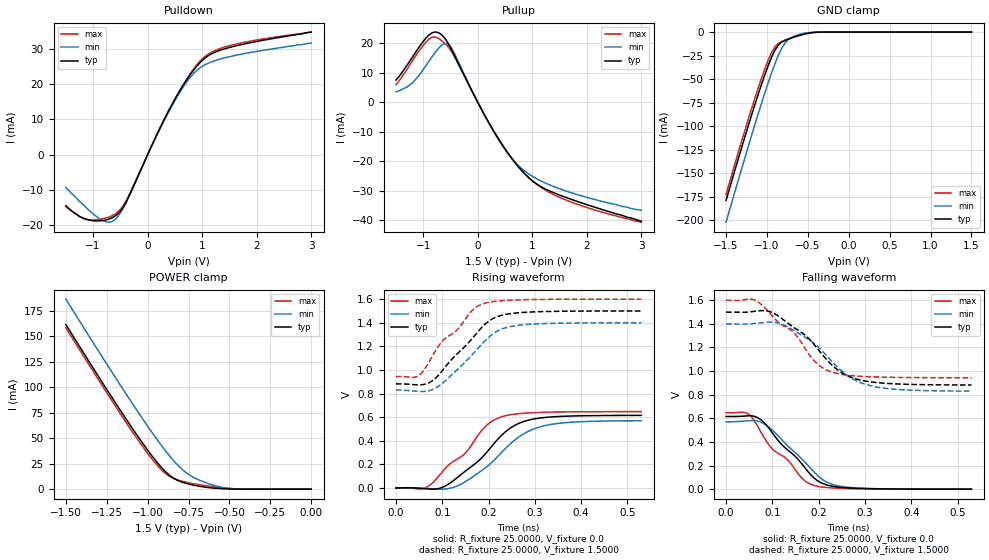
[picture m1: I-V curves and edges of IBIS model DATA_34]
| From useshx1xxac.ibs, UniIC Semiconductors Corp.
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|When TDQS is enabled, NU_TDQS is a output with terminal resistance;
|When TDQS is disabled, NU_TDQS is a DM;
|   Model DATA_34
[Model]  DATA_34
Model_type   I/O
Polarity   Non-Inverting
Enable   Active-High
Vinl =   0.600000V
Vinh =   0.900000V
Vmeas =   0.750000V
Rref =   25.0000000
Vref =   0.7500000V
C_comp   1.3900pF   1.3640pF   1.5600pF
[Temperature Range]   25.0000   95.0000   0.0
[Voltage Range]   1.5000V   1.4000V   1.6000V
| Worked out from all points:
|   slope of the pulldown table from 0 to 0.225 V, typ, clamps not added: 29.8 ohm
|   slope of the pullup table from 0 to 0.225 V, typ, clamps not added: 29.6 ohm
|   GND clamp passes 1 mA (typ) near -0.48 V on its own axis
|   POWER clamp passes 1 mA (typ) near -0.59 V on its own axis
|   rising waveform, R_fixture 25.0000, V_fixture 0.0: 20-80 % time 98.2ps typ, 102ps min, 94ps max; typ from 0 V to 0.615 V
|   rising waveform, R_fixture 25.0000, V_fixture 1.5000: 20-80 % time 86.9ps typ, 86.6ps min, 84.5ps max; typ from 0.882 V to 1.5 V
|   falling waveform, R_fixture 25.0000, V_fixture 0.0: 20-80 % time 85.5ps typ, 86.9ps min, 85.6ps max; typ from 0.615 V to 0 V
|   falling waveform, R_fixture 25.0000, V_fixture 1.5000: 20-80 % time 99ps typ, 99.1ps min, 94.3ps max; typ from 1.5 V to 0.882 V
[Pulldown]
|Voltage   I(typ)   I(min)   I(max)
-1.5V     -14.6mA    -9.3mA     -14.4mA
-1.1V     -18.42mA   -15.42mA   -18.46mA
-850mV    -18.72mA   -18.45mA   -18.26mA
-650mV    -17.88mA   -18.95mA   -17.28mA
-550mV    -16.86mA   -17.64mA   -16.27mA
-400mV    -13.69mA   -13.63mA   -13.24mA
400mV     12.93mA    12.56mA    12.74mA
700mV     20.91mA    20.27mA    20.98mA
900mV     25.09mA    23.93mA    25.48mA
1.1V      27.97mA    25.89mA    28.43mA
1.4V      30mA       27.43mA    30.5mA
3V        34.8mA     31.7mA     34.8mA
[Pullup]
|Voltage   I(typ)   I(min)   I(max)
-1.5V     7.5mA      3.5mA      5.9mA
-1.2V     15.18mA    6.5mA      13.95mA
-850mV    23.36mA    15.05mA    21.87mA
-700mV    23.33mA    18.57mA    21.38mA
-550mV    20.17mA    19.79mA    18.86mA
-450mV    16.69mA    17.37mA    16.22mA
300mV     -9.979mA   -10.24mA   -9.941mA
550mV     -17.14mA   -17.23mA   -17.11mA
800mV     -23mA      -22.34mA   -23.02mA
1.1V      -27.91mA   -26.09mA   -28.08mA
1.55V     -31.76mA   -29.61mA   -32.58mA
3V        -40.3mA    -36.6mA    -40.6mA
[GND_clamp]
|Voltage   I(typ)   I(min)   I(max)
-1.5V     -178.7mA   -201.8mA   -172.1mA
-1.18V    -85.9mA    -107.5mA   -79.02mA
-1.06V    -53.85mA   -73.82mA   -47.38mA
-980mV    -34.46mA   -52.52mA   -28.79mA
-940mV    -25.94mA   -42.47mA   -21.09mA
-900mV    -18.8mA    -33.04mA   -15.34mA
-860mV    -13.68mA   -24.5mA    -11.91mA
-780mV    -8.804mA   -11.75mA   -8.617mA
-740mV    -7.413mA   -8.071mA   -7.384mA
-620mV    -3.934mA   -2.917mA   -4.046mA
-420mV    -302.4uA   -187.9uA   -428.5uA
1.5V      1.623nA    17.64nA    1.98nA
[POWER_clamp]
|Voltage   I(typ)   I(min)   I(max)
-1.5V     161.3mA    186.3mA    158.3mA
-1.22V    90.37mA    115.2mA    87.1mA
-1.04V    47.2mA     71.18mA    43.94mA
-980mV    33.96mA    57.17mA    30.91mA
-920mV    22.07mA    43.79mA    19.67mA
-880mV    15.49mA    35.42mA    14.07mA
-840mV    10.61mA    27.72mA    10.46mA
-780mV    6.409mA    18.15mA    7.405mA
-720mV    3.991mA    11.66mA    5.381mA
-560mV    586.1uA    2.318mA    1.645mA
-440mV    47uA       184.9uA    218uA
0V        1.623nA    5.301nA    2.263nA
[Ramp]
| variable   typ   min   max
dV/dt_r  0.3694/99.9524p   0.3422/0.1029n   0.3883/95.3273p
dV/dt_f  0.3712/0.1005n   0.3425/0.1006n   0.3941/95.4886p
R_load = 25.0000
[Rising Waveform]
R_fixture= 25.0000
V_fixture= 0.0
V_fixture_min= 0.0
V_fixture_max= 0.0
|time   V(typ)   V(min)   V(max)
0s        0V         0V         0V
65ps      -6.55mV    -3.923mV   2.939mV
105ps     13.96mV    -8.608mV   159.8mV
155ps     158.2mV    66.17mV    319.3mV
195ps     297.2mV    176.3mV    527.8mV
230ps     452.9mV    308.8mV    605mV
275ps     561.8mV    456.7mV    632.8mV
325ps     598.4mV    531mV      641.6mV
395ps     611.1mV    560.7mV    645.4mV
530ps     615.1mV    569.3mV    646.9mV
[Rising Waveform]
R_fixture= 25.0000
V_fixture= 1.5000
V_fixture_min= 1.4000
V_fixture_max= 1.6000
|time   V(typ)   V(min)   V(max)
0s        882.1mV    830.4mV    943.5mV
45ps      874mV      819mV      942.7mV
75ps      898.8mV    827.8mV    1.091V
100ps     992.8mV    885.7mV    1.243V
130ps     1.127V     993.3mV    1.331V
170ps     1.29V      1.151V     1.522V
190ps     1.378V     1.236V     1.562V
225ps     1.459V     1.341V     1.585V
265ps     1.484V     1.378V     1.593V
530ps     1.5V       1.4V       1.6V
[Falling Waveform]
R_fixture= 25.0000
V_fixture= 0.0
V_fixture_min= 0.0
V_fixture_max= 0.0
|time   V(typ)   V(min)   V(max)
0s        615.1mV    569.3mV    646.9mV
45ps      620.4mV    578.5mV    643.7mV
75ps      588.4mV    567.5mV    485.2mV
100ps     477.1mV    500.9mV    340.4mV
130ps     342.3mV    379.5mV    259.7mV
170ps     182.8mV    230.5mV    71.02mV
190ps     94.3mV     146.2mV    31.84mV
220ps     32.85mV    55.49mV    13.08mV
260ps     11.35mV    17.37mV    5.508mV
530ps     0V         0V         0V
[Falling Waveform]
R_fixture= 25.0000
V_fixture= 1.5000
V_fixture_min= 1.4000
V_fixture_max= 1.6000
|time   V(typ)   V(min)   V(max)
0s        1.5V       1.4V       1.6V
60ps      1.506V     1.403V     1.605V
100ps     1.496V     1.414V     1.465V
145ps     1.373V     1.348V     1.331V
180ps     1.27V      1.263V     1.136V
200ps     1.178V     1.201V     1.051V
230ps     1.046V     1.075V     990.2mV
270ps     948mV      943mV      962.1mV
320ps     905mV      869.1mV    950.7mV
530ps     882.1mV    830.4mV    943.5mV
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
